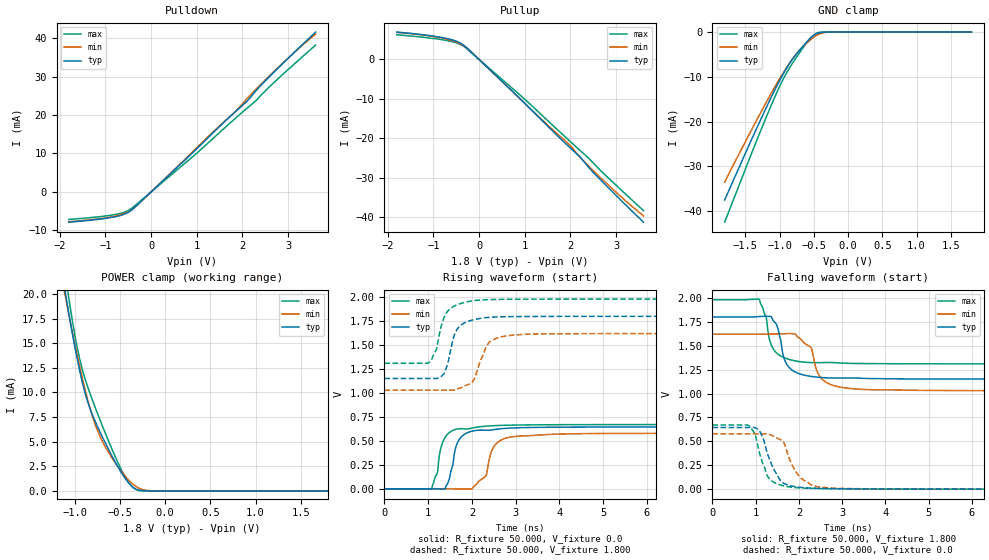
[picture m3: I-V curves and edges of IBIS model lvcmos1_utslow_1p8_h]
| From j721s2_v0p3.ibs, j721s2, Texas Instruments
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|   utslow_1p8_h
[Model]   lvcmos1_utslow_1p8_h
Model_type I/O
Polarity   Non-Inverting
Enable   Active-High
Vinl = 0
Vinh = 0.8
Vmeas = 0.9
Vref = 1.8
Cref = 2pF
Rref = 100000
|   typ   min   max
C_comp   2.761pF   2.531pF   2.966pF
[Voltage Range]   1.8   1.62   1.98
[Temperature Range]   27   150   -40
[Pullup Reference]   1.8   1.62   1.98
[Pulldown Reference]   0   0   0
[Power Clamp Reference]   1.8   1.62   1.98
[GND Clamp Reference]   0   0   0
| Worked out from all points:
|   slope of the pulldown table from 0 to 0.27 V, typ, clamps not added: 89.4 ohm
|   slope of the pullup table from 0 to 0.27 V, typ, clamps not added: 90.5 ohm
|   GND clamp passes 1 mA (typ) near -0.52 V on its own axis
|   POWER clamp passes 1 mA (typ) near -0.42 V on its own axis
|   rising waveform, R_fixture 50.000, V_fixture 0.0: 20-80 % time 217ps typ, 264ps min, 212ps max; typ from 0 V to 0.645 V
|   rising waveform, R_fixture 50.000, V_fixture 1.800: 20-80 % time 241ps typ, 300ps min, 256ps max; typ from 1.15 V to 1.8 V
|   falling waveform, R_fixture 50.000, V_fixture 1.800: 20-80 % time 238ps typ, 329ps min, 249ps max; typ from 1.8 V to 1.15 V
|   falling waveform, R_fixture 50.000, V_fixture 0.0: 20-80 % time 337ps typ, 376ps min, 270ps max; typ from 0.645 V to 0 V
[Pulldown]
|Voltage   I(typ)   I(min)   I(max)
-1.8V     -7.878mA   -7.741mA   -7.164mA
-1.194V   -7.199mA   -7.066mA   -6.526mA
-808mV    -6.535mA   -6.343mA   -5.925mA
-588mV    -5.811mA   -5.63mA    -5.299mA
-422mV    -4.67mA    -4.628mA   -4.233mA
-257mV    -2.879mA   -2.941mA   -2.588mA
955mV     10.71mA    10.96mA    9.612mA
1.837V    20.75mA    20.83mA    19.06mA
2.057V    23.12mA    23.66mA    21.35mA
2.278V    26.05mA    26.5mA     23.54mA
2.773V    32.13mA    32.27mA    29.36mA
3.6V      41.56mA    41.06mA    38.17mA
[Pullup]
|Voltage   I(typ)   I(min)   I(max)
-1.8V     6.924mA    6.85mA     6.245mA
-1.194V   6.205mA    6.128mA    5.571mA
-753mV    5.423mA    5.26mA     4.889mA
-478mV    4.524mA    4.309mA    4.114mA
-312mV    3.403mA    3.276mA    3.122mA
1.01V     -11.23mA   -11.23mA   -10.18mA
1.947V    -21.88mA   -21.25mA   -20.26mA
2.222V    -24.84mA   -24.92mA   -23.17mA
2.443V    -27.9mA    -27.51mA   -25.54mA
2.718V    -31.18mA   -30.61mA   -28.78mA
3.214V    -36.9mA    -35.87mA   -34.18mA
3.6V      -41.23mA   -39.63mA   -38.29mA
[GND_clamp]
|Voltage   I(typ)   I(min)   I(max)
-1.8V     -37.5mA    -33.49mA   -42.48mA
-1.318V   -20.97mA   -19.21mA   -23.65mA
-1.132V   -14.92mA   -13.99mA   -16.76mA
-984mV    -10.42mA   -10.06mA   -11.66mA
-872mV    -7.441mA   -7.36mA    -8.464mA
-761mV    -5.054mA   -4.998mA   -5.817mA
-687mV    -3.665mA   -3.691mA   -4.162mA
-575mV    -1.732mA   -2.058mA   -1.807mA
-501mV    -715.1uA   -1.141mA   -632.9uA
-427mV    -156.5uA   -468.3uA   -83.58uA
-278mV    -1.298uA   -23.76uA   -249.6nA
1.8V      0A         0A         0A
[POWER_clamp]
|Voltage   I(typ)   I(min)   I(max)
-1.8V     63.27mA    56.65mA    71.18mA
-1.095V   19.71mA    19.39mA    21.45mA
-1.058V   17.7mA     17.64mA    19.19mA
-984mV    13.96mA    14.3mA     15.13mA
-946mV    12.29mA    12.72mA    13.48mA
-872mV    9.525mA    9.826mA    11mA
-761mV    6.814mA    6.466mA    8.201mA
-649mV    4.665mA    4.295mA    5.607mA
-464mV    1.579mA    1.755mA    1.805mA
-315mV    157.8uA    414.1uA    109uA
-130mV    309.5nA    7.644uA    148.4nA
1.8V      0A         0A         0A
[Ramp]
| variable   typ   min   max
dV/dt_r   0.387/0.216n   0.347/0.262n   0.402/0.212n
dV/dt_f   0.389/0.237n   0.355/0.329n   0.402/0.249n
R_load = 50.000
[Rising Waveform]
R_fixture= 50.000
V_fixture= 0.0
V_fixture_min= 0.0
V_fixture_max= 0.0
|time   V(typ)   V(min)   V(max)
0s        971.9nV    20.68uV    1.71uV
1.075ns   146.5uV    21.15uV    -2.46mV
1.388ns   2.093mV    60.95uV    537.2mV
1.489ns   111.7mV    -112.2uV   588.4mV
1.663ns   474.1mV    -1.716mV   623.7mV
1.992ns   599.8mV    -1.51mV    632.1mV
2.286ns   611.7mV    118.2mV    652mV
2.503ns   617.2mV    440.1mV    658.5mV
2.913ns   634mV      542.4mV    664.3mV
10ns      644.8mV    578.7mV    670.4mV
[Rising Waveform]
R_fixture= 50.000
V_fixture= 1.800
V_fixture_min= 1.620
V_fixture_max= 1.980
|time   V(typ)   V(min)   V(max)
0s        1.151V     1.029V     1.31V
1.005ns   1.151V     1.029V     1.314V
1.19ns    1.151V     1.029V     1.457V
1.315ns   1.179V     1.029V     1.725V
1.433ns   1.285V     1.029V     1.845V
1.632ns   1.641V     1.036V     1.914V
2.019ns   1.762V     1.122V     1.962V
2.373ns   1.788V     1.515V     1.974V
2.837ns   1.796V     1.599V     1.978V
10ns      1.8V       1.62V      1.98V
[Falling Waveform]
R_fixture= 50.000
V_fixture= 1.800
V_fixture_min= 1.620
V_fixture_max= 1.980
|time   V(typ)   V(min)   V(max)
0s        1.8V       1.62V      1.98V
1.08ns    1.805V     1.62V      1.985V
1.363ns   1.802V     1.622V     1.506V
1.517ns   1.678V     1.622V     1.411V
1.692ns   1.329V     1.625V     1.368V
2.005ns   1.207V     1.58V      1.334V
2.282ns   1.179V     1.478V     1.323V
2.507ns   1.168V     1.165V     1.323V
2.976ns   1.161V     1.065V     1.318V
10ns      1.151V     1.029V     1.31V
[Falling Waveform]
R_fixture= 50.000
V_fixture= 0.0
V_fixture_min= 0.0
V_fixture_max= 0.0
|time   V(typ)   V(min)   V(max)
0s        644.8mV    578.8mV    670.4mV
829ps     644.8mV    578.8mV    668.2mV
983ps     643.4mV    578.8mV    578.5mV
1.053ns   625.8mV    578.8mV    447.8mV
1.301ns   336mV      574.4mV    119mV
1.626ns   68.15mV    500.3mV    37.21mV
1.786ns   38.1mV     310.1mV    23.22mV
2.073ns   17.08mV    106.6mV    12.07mV
2.625ns   6.449mV    15.76mV    5.342mV
10ns      39.48uV    98.51uV    21.99uV
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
